PROGRAM MAIN
VAR
	fbProxyConvert	: FB_DynProxyTcComConvertModule(	classID		:= STRING_TO_GUID('f229f89c-d59b-4036-b41f-784807c6fb38'),
														IID			:= TC_GLOBAL_IID_LIST.IID_IAnalogToPWM,
														sObjectName	:= 'DataConvertDrv:fbProxyConvert',
														eObjState   := TCOM_STATE.TCOM_STATE_OP);
	AnalogValue		: LREAL	:= 50;
	bPwmPos			: BOOL;
	bPwmNeg			: BOOL;
	TestCounter		: DINT;
	INITED			: BOOL	:= FALSE;
	binit			: BOOL;	
	
	hr				: HRESULT;

	bChange			: BOOL;
	bDelete			: BOOL;
	bExecute		: BOOL;
END_VAR



IF fbProxyConvert.ip <> 0 THEN

	fbProxyConvert.Cyclic();

	IF  binit THEN
		fbProxyConvert.ip.initParam(T#1S);
		binit:=FALSE;
		INITED:= TRUE;
	END_IF

	IF bExecute THEN
		hr := fbProxyConvert.ip.Convert(AnalogValue,ADR(bPwmPos),ADR(bPwmNeg),ADR(TestCounter));
	END_IF
	
	IF bChange THEN
		hr := fbProxyConvert.iTcComobject.TcSetObjState(TCOM_STATE.TCOM_STATE_PREOP,fbProxyConvert.iTComObjectServer,0);
	END_IF
END_IF


IF bDelete THEN
	fbProxyConvert.FB_exit(FALSE);
	bDelete:= FALSE;
END_IF

END_PROGRAM
